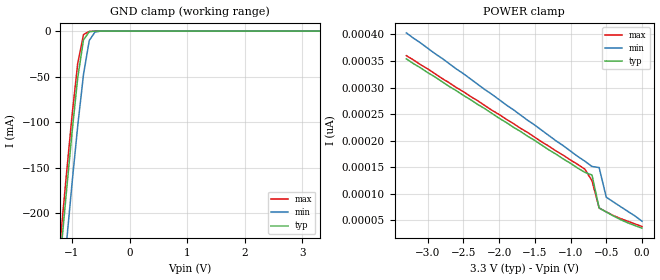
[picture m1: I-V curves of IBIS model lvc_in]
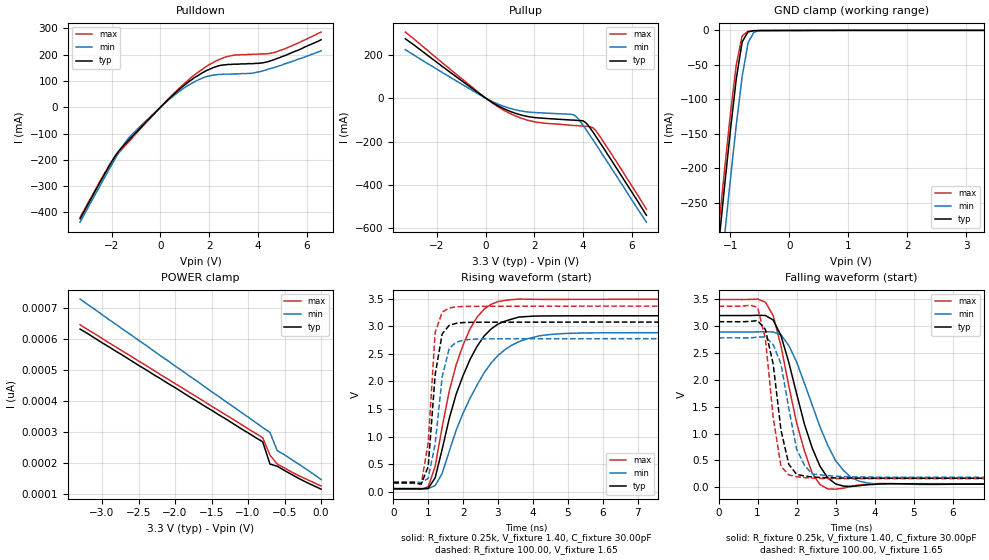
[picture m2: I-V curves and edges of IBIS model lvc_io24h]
| IBIS file 32245xh.ibs created by s2ibis2 version 1.1
| North Carolina State University Electronics Research Laboratory  1995
[IBIS ver]   2.1
[File name]   32245xh.ibs
[File Rev]   1.0
[Date]   03/01/99
[Source]   Integrated Device Technology, Inc.
[Notes]   1.Temperatures: typ=25C, min=100C, max=0C 2.RRmp rates based
   on 50 ohm load.
[Disclaimer] Integrated Device Technology, Inc. ("IDT") hereby grants the
   user of this IBIS model a non-exclusive, nontransferable
   license to use this IBIS model under the following terms. The
   user is granted this license only to use the IBIS model and is
   not granted rights to sell, copy (except as needed to run the
   IBIS model), rent, lease or sub-license the IBIS model in
   whole or in part, or in modified form to anyone. The User may
   modify the IBIS model to suit its specific applications, but
   rights to derivative works and such modifications shall belong
   to IDT. This IBIS model is provided on an AS IS" basis and IDT
   makes absolutely no warranty with respect to the information
   contained herein. IDT DISCLAIMS AND CUSTOMER WAIVES ALL
   WARRANTIES, EXPRESS AND IMPLIED, INCLUDING WARRANTIES OF
   MERCHANTABILITY AND FITNESS FOR A PARTICULAR PURPOSE. THE
   ENTIRE RISK AS TO QUALITY AND PERFORMANCE IS WITH THE USER
   ACCORDINGLY, IN NO EVENT SHALL IDT BE LIABLE FOR ANY DIRECT OR
   INDIRECT DAMAGES, WHETHER IN CONTRACT OR TORT, INCLUDING ANY
   LOST PROFITS OR OTHER INCIDENTAL, CONSEQUENTIAL, EXEMPLARY, OR
   PUNITIVE DAMAGES ARISING OUT OF THE USE OR APPLICATION OF THE
   IBIS model. Further, IDT reserves the right to make changes
   without notice to any product herein to improve reliability,
   function, or design. IDT does not convey any license under
   patent rights or any other intellectual property rights,
   including those of third parties. IDT is not obligated to
   provide maintenance or support for the licensed IBIS model.
[Copyright]   Copyright 1997, Integrated Device Technology, Inc. all rights
   reserved
|   Component LVCH32245
[Component]   LVCH32245
[Manufacturer]   Integrated Device Technology
[Package]
| BF96
| variable   typ   min   max
R_pkg   144.3m   NA   NA
L_pkg   4.10nH   NA   NA
C_pkg   0.36pF   NA   NA
[Pin]  signal_name   model_name   R_pin   L_pin   C_pin
A1   1B2   lvc_io24h
A2   1B1   lvc_io24h
A3   1DIR   lvc_in
A4   1OEB   lvc_in
A5   1A1   lvc_io24h
A6   1A2   lvc_io24h
B1   1B4   lvc_io24h
B2   1B3   lvc_io24h
B3   GND   GND
B4   GND   GND
B5   1A3   lvc_io24h
B6   1A4   lvc_io24h
C1   1B6   lvc_io24h
C2   1B5   lvc_io24h
C3   VCC   POWER
C4   VCC   POWER
C5   1A5   lvc_io24h
C6   1A6   lvc_io24h
D1   1B8   lvc_io24h
D2   1B7   lvc_io24h
D3   GND   GND
D4   GND   GND
D5   1A7   lvc_io24h
D6   1A8   lvc_io24h
E1   2B2   lvc_io24h
E2   2B1   lvc_io24h
E3   GND   GND
E4   GND   GND
E5   2A1   lvc_io24h
E6   2A2   lvc_io24h
F1   2B4   lvc_io24h
F2   2B3   lvc_io24h
F3   VCC   POWER
F4   VCC   POWER
F5   2A3   lvc_io24h
F6   2A4   lvc_io24h
G1   2B6   lvc_io24h
G2   2B5   lvc_io24h
G3   GND   GND
G4   GND   GND
G5   2A5   lvc_io24h
G6   2A6   lvc_io24h
H1   2B7   lvc_io24h
H2   2B8   lvc_io24h
H3   2DIR   lvc_in
H4   2OEB   lvc_in
H5   2A8   lvc_io24h
H6   2A7   lvc_io24h
J1   3B2   lvc_io24h
J2   3B1   lvc_io24h
J3   3DIR   lvc_in
J4   3OEB   lvc_in
J5   3A1   lvc_io24h
J6   3A2   lvc_io24h
K1   3B4   lvc_io24h
K2   3B3   lvc_io24h
K3   GND   GND
K4   GND   GND
K5   3A3   lvc_io24h
K6   3A4   lvc_io24h
L1   3B6   lvc_io24h
L2   3B5   lvc_io24h
L3   VCC   POWER
L4   VCC   POWER
L5   3A5   lvc_io24h
L6   3A6   lvc_io24h
M1   3B8   lvc_io24h
M2   3B7   lvc_io24h
M3   GND   GND
M4   GND   GND
M5   3A7   lvc_io24h
M6   3A8   lvc_io24h
N1   4B2   lvc_io24h
N2   4B1   lvc_io24h
N3   GND   GND
N4   GND   GND
N5   4A1   lvc_io24h
N6   4A2   lvc_io24h
P1   4B4   lvc_io24h
P2   4B3   lvc_io24h
P3   VCC   POWER
P4   VCC   POWER
P5   4A3   lvc_io24h
P6   4A4   lvc_io24h
R1   4B6   lvc_io24h
R2   4B5   lvc_io24h
R3   GND   GND
R4   GND   GND
R5   4A5   lvc_io24h
R6   4A6   lvc_io24h
T1   4B7   lvc_io24h
T2   4B8   lvc_io24h
T3   4DIR   lvc_in
T4   4OEB   lvc_in
T5   4A8   lvc_io24h
T6   4A7   lvc_io24h
| Models and submodels in the file (2): lvc_in (Input), lvc_io24h (I/O)
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| in   in   dummy_model
| oe   oe
|   Model lvc_in
[Model]   lvc_in
Model_type   Input
Vinl =  0.800V
Vinh =  2.000V
C_comp   3.00pF   NA   NA
[Temperature Range]   25.00   100.00   0.000
[Voltage Range]   3.30V   3.00V   3.60V
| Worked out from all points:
|   GND clamp passes 1 mA (typ) near -0.70 V on its own axis
[GND_clamp]
| voltage   I(typ)   I(min)   I(max)
-3.3V     -1.806A    -1.858A    -1.789A
-1.2V     -248mA     -306mA     -229mA
-1.1V     -179mA     -236mA     -160mA
-1V       -112mA     -168mA     -93.56mA
-900mV    -51.39mA   -104mA     -35.36mA
-800mV    -9.697mA   -47.7mA    -3.786mA
-700mV    -714uA     -10.4mA    -348uA
-600mV    -52.42uA   -951uA     -8.225uA
-500mV    -126nA     -30.48uA   -10.89nA
3.3V      34.69pA    75.27pA    23pA
[POWER_clamp]
| voltage   I(typ)   I(min)   I(max)
-3.3V     354pA      403pA      360pA
-800mV    140pA      161pA      146pA
-700mV    135pA      151pA      124pA
-600mV    72.75pA    149pA      72.79pA
-500mV    65.09pA    93.05pA    65.39pA
-300mV    50.77pA    75.27pA    52.78pA
0V        34.68pA    47.91pA    37.83pA
|   Model lvc_io24h
[Model]   lvc_io24h
Model_type   I/O
Polarity   Non-Inverting
Enable   Active-High
Vinl =  0.000V
Vinh =  2.000V
Vmeas =  1.500V
C_comp   3.00pF   NA   NA
[Temperature Range]   25.00   100.00   0.000
[Voltage Range]   3.30V   3.00V   3.60V
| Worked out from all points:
|   slope of the pulldown table from 0 to 0.495 V, typ, clamps not added: 11.1 ohm
|   slope of the pullup table from 0 to 0.495 V, typ, clamps not added: 14.5 ohm
|   GND clamp passes 1 mA (typ) near -0.64 V on its own axis
|   rising waveform, R_fixture 0.25k, V_fixture 1.40, C_fixture 30.00pF: 20-80 % time 974ps typ, 1.24ns min, 819ps max; typ from 0.061 V to 3.19 V
|   rising waveform, R_fixture 100.00, V_fixture 1.65: 20-80 % time 266ps typ, 323ps min, 208ps max; typ from 0.171 V to 3.08 V
|   falling waveform, R_fixture 0.25k, V_fixture 1.40, C_fixture 30.00pF: 20-80 % time 725ps typ, 902ps min, 639ps max; typ from 3.19 V to 0.061 V
|   falling waveform, R_fixture 100.00, V_fixture 1.65: 20-80 % time 362ps typ, 397ps min, 304ps max; typ from 3.08 V to 0.171 V
[Pulldown]
| voltage   I(typ)   I(min)   I(max)
-3.3V     -424mA     -437mA     -419mA
-2.1V     -223mA     -235mA     -220mA
-1.8V     -177mA     -186mA     -182mA
-1.4V     -135mA     -128mA     -141mA
47.68nV   4.51nA     4.11nA     4.76nA
900mV     77.7mA     68.8mA     83.4mA
1.8V      135mA      114mA      150mA
2.6V      161mA      126mA      189mA
3.7V      166mA      129mA      201mA
4.4V      173mA      144mA      204mA
5.1V      196mA      165mA      222mA
6.6V      257mA      215mA      286mA
[Pullup]
| voltage   I(typ)   I(min)   I(max)
-3.3V     273mA      223mA      304mA
-200mV    15.7mA     12.6mA     17.8mA
800mV     -51.2mA    -39.9mA    -59.2mA
1.4V      -75.9mA    -58mA      -89.7mA
2V        -89.2mA    -66.1mA    -109mA
3.5V      -101mA     -74.3mA    -125mA
3.7V      -102mA     -83mA      -126mA
4.1V      -112mA     -141mA     -130mA
4.4V      -155mA     -191mA     -136mA
4.5V      -172mA     -208mA     -147mA
5.2V      -292mA     -329mA     -263mA
6.6V      -539mA     -571mA     -511mA
[GND_clamp]
| voltage   I(typ)   I(min)   I(max)
-3.3V     -2.217A    -2.283A    -2.195A
-1.2V     -312mA     -384mA     -288mA
-1.1V     -227mA     -299mA     -203mA
-1V       -145mA     -216mA     -121mA
-900mV    -69.9mA    -137mA     -49.49mA
-800mV    -16.48mA   -66.49mA   -7.75mA
-700mV    -2.021mA   -17.86mA   -1.171mA
-600mV    -313uA     -2.437mA   -215uA
-500mV    -136uA     -188uA     -155uA
3.3V      163uA      116uA      211uA
[POWER_clamp]
| voltage   I(typ)   I(min)   I(max)
-3.3V     631pA      728pA      645pA
-800mV    267pA      313pA      280pA
-700mV    195pA      297pA      224pA
-600mV    188pA      238pA      195pA
-300mV    148pA      194pA      157pA
0V        114pA      145pA      124pA
[Ramp]
| variable   typ   min   max
dV/dt_r   1.45/0.32n   1.21/0.34n   1.64/0.23n
dV/dt_f   1.59/0.39n   1.41/0.50n   1.76/0.35n
R_load = 50.00
[Rising Waveform]
R_fixture = 0.25k
V_fixture = 1.40
C_fixture = 30.00pF
R_dut = 7.00m
L_dut = 3.30nH
C_dut = 0.29pF
| time   V(typ)   V(min)   V(max)
0s        61.18mV    67.45mV    57.75mV
1ns       68.22mV    64.57mV    94.91mV
1.2ns     260mV      117mV      469mV
1.4ns     775mV      340mV      1.176V
1.6ns     1.324V     733mV      1.82V
2ns       2.108V     1.429V     2.659V
2.4ns     2.635V     1.936V     3.163V
3ns       3.038V     2.47V      3.444V
5ns       3.187V     2.869V     3.484V
19.8ns    3.189V     2.884V     3.487V
[Rising Waveform]
R_fixture = 100.00
V_fixture = 1.65
R_dut = 7.00m
L_dut = 3.30nH
C_dut = 0.29pF
| time   V(typ)   V(min)   V(max)
0s        171mV      188mV      161mV
800ps     147mV      174mV      143mV
1ns       463mV      248mV      895mV
1.2ns     2.124V     874mV      2.888V
1.4ns     2.86V      2.079V     3.252V
1.6ns     3.014V     2.598V     3.329V
1.8ns     3.052V     2.708V     3.35V
2ns       3.065V     2.747V     3.356V
2.6ns     3.071V     2.77V      3.359V
19.8ns    3.075V     2.775V     3.362V
[Falling Waveform]
R_fixture = 0.25k
V_fixture = 1.40
C_fixture = 30.00pF
R_dut = 7.00m
L_dut = 3.30nH
C_dut = 0.29pF
| time   V(typ)   V(min)   V(max)
0s        3.189V     2.884V     3.487V
1ns       3.194V     2.885V     3.495V
1.4ns     3.106V     2.884V     3.187V
1.8ns     2.32V      2.633V     1.883V
2.2ns     1.176V     1.933V     680mV
2.4ns     732mV      1.53V      262mV
2.8ns     175mV      780mV      -28.91mV
3.4ns     17.82mV    181mV      19.19mV
4ns       57.02mV    65.71mV    68.19mV
19.8ns    61.19mV    67.46mV    57.75mV
[Falling Waveform]
R_fixture = 100.00
V_fixture = 1.65
R_dut = 7.00m
L_dut = 3.30nH
C_dut = 0.29pF
| time   V(typ)   V(min)   V(max)
0s        3.075V     2.775V     3.362V
1ns       3.095V     2.788V     3.342V
1.2ns     2.931V     2.794V     2.759V
1.4ns     2.285V     2.647V     1.295V
1.6ns     1.061V     2.291V     390mV
1.8ns     428mV      1.467V     231mV
2ns       243mV      713mV      198mV
2.4ns     193mV      248mV      172mV
3.2ns     174mV      201mV      163mV
19.8ns    171mV      188mV      161mV
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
